FUNCTION_BLOCK "Function Block"
	VAR_INPUT
		INVAR : S5TIME;
	END_VAR
BEGIN
	NOP		0
END_FUNCTION_BLOCK


DATA_BLOCK "Data_1"
STRUCT
	VAR0		: INT;
END_STRUCT;
BEGIN
	VAR0		:= 123;
END_DATA_BLOCK


DATA_BLOCK "Instance DB"
	"Function Block"
BEGIN
END_DATA_BLOCK


ORGANIZATION_BLOCK OB 1
BEGIN
	// Test symbolic M access
	__STWRST
	U		"sym_M_0.0"
	__ASSERT==	__STW VKE,	0
	SET
	=		M 0.0
	__STWRST
	U		"sym_M_0.0"
	__ASSERT==	__STW VKE,	1
	CLR
	=		"sym_M_0.0"
	__STWRST
	U		M 0.0
	__ASSERT==	__STW VKE,	0


	// Test symbolic fully qualified access
	L		"Data_1".VAR0
	__ASSERT==	__ACCU 1,	123


	// Test symbolic FB call
	CALL	"Function Block", "Instance DB" (
		INVAR := 100,
	)


	// Test symbolic timer/counter access
	CLR
	SI		"symbolic timer"
	U		"symbolic timer"
	=		M 0.0
	CLR
	ZR		"symbolic counter"
	U		"symbolic counter"
	=		M 0.0


	CALL SFC 46 // STOP CPU
END_ORGANIZATION_BLOCK
